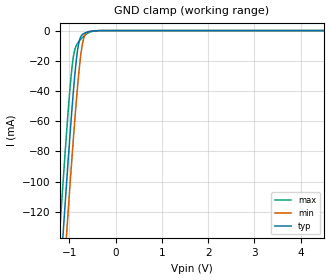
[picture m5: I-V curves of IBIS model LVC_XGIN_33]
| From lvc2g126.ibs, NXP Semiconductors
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|   Model LVC_XGIN_33
[Model]   LVC_XGIN_33
Model_type   Input
Vinl =   0.8V
Vinh =   2.0V
C_comp   2.96pF   2.12pF   3.91pF
[Model Spec]
| Note: The input and output voltage ratings may be exceeded if the input and
|   output current ratings are observed (please refer to the data sheet)
|   Subparameter   typ   min   max
| Thresholds
Vinh   2.0   2.0   2.0
Vinl   0.8   0.8   0.8
| Overshoot
S_overshoot_high   6.5   6.5   6.5   | Static overshoot
S_overshoot_low   -0.5   -0.5   -0.5
D_overshoot_high   7.2   7.2   7.2   | Dynamic overshoot
D_overshoot_low   -0.95   -0.9   -1.0
D_overshoot_time   3n   3n   3n
|Ambient temperature:   25   85   -40
[Temperature Range]   50   105   -10
[Voltage Range]   3.3V   3.0V   3.6V
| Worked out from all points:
|   GND clamp passes 1 mA (typ) near -0.61 V on its own axis
|Process Range   nominal   slow   fast
[GND_clamp]
| voltage   I(typ)   I(min)   I(max)
-5.5V     -2.277A    -2.307A    -2.246A
-1.221V   -173.6mA   -208.2mA   -138.8mA
-1.2V     -163.7mA   -198.3mA   -129mA
-1.136V   -134.3mA   -168.7mA   -99.82mA
-1.071V   -105.4mA   -139.6mA   -71.73mA
-1.05V    -95.98mA   -130mA     -62.73mA
-942.9mV  -51.21mA   -83.48mA   -24.05mA
-900mV    -35.22mA   -65.87mA   -14.8mA
-835.7mV  -15.71mA   -41.31mA   -9.021mA
-728.6mV  -2.901mA   -10.64mA   -4.899mA
-642.9mV  -1.321mA   -1.88mA    -2.576mA
5.5V      0A         0A         0A
